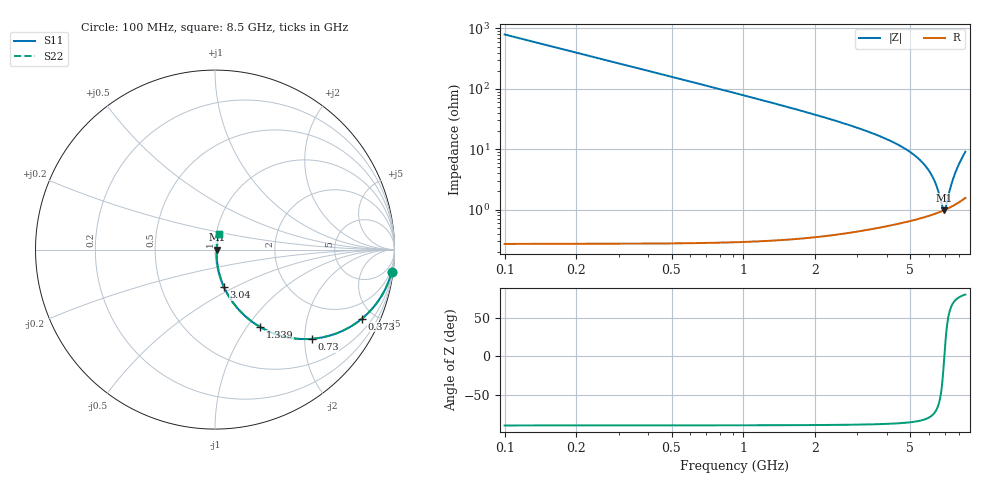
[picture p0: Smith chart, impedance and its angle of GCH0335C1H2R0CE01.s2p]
!Murata Part Number: GCH0335C1H2R0CE01
!These Parameters are Measured in Series Mode Connection
!Data Generated on Mar 13, 2026
!  o--ll--o
!Port1  Port2
!  o------o
!Operation Temp=25[degC], DC Bias Voltage=0[V]
!Freq. Start=100[MHz] Stop=9[GHz] 401[Steps]
# Hz S RI R 50
!Freq.(Hz) S11(Real) S11(Imag) S21(Real) S21(Imag) S12(Real) S12(Imag) S22(Real) S22(Imag)
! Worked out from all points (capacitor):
!   401 points, 100 MHz to 8.5 GHz, reference 50 ohm
!   read as one part in series: C = 2 pF near 142 MHz
!   lowest |Z| = 979 mohm at 6.925 GHz (marker M1)
!   series resonance near 6.94 GHz, so ESL is about 260 pH
!   S11 on the Smith chart (normalised r, x): 100 MHz: 1, -16; 373 MHz: 1.01, -4.26; 730 MHz: 1.01, -2.16; 1.339 GHz: 1.01, -1.15; 3.04 GHz: 1.01, -0.44; 8.5 GHz: 1.03, +0.18
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1e8  0.9844 -0.1237  0.0156 0.1237  0.0156 0.1237  0.9844 -0.1237
2.26e8  0.9251 -0.2629  0.0749 0.2629  0.0749 0.2629  0.9251 -0.2629
3.73e8  0.8189 -0.3845  0.1811 0.3845  0.1811 0.3845  0.8189 -0.3845
5.41e8  0.6816 -0.4649  0.3184 0.4649  0.3184 0.4649  0.6816 -0.4649
7.3e8  0.5387 -0.4972  0.4613 0.4972  0.4613 0.4972  0.5387 -0.4972
1.024e9  0.3691 -0.4807  0.6309 0.4807  0.6309 0.4807  0.3691 -0.4807
1.339e9  0.2511 -0.431  0.7489 0.431  0.7489 0.431  0.2511 -0.431
1.507e9  0.2072 -0.4022  0.7928 0.4022  0.7928 0.4022  0.2072 -0.4022
2.095e9  0.1133 -0.312  0.8867 0.312  0.8867 0.312  0.1133 -0.312
2.914e9  0.0561 -0.2212  0.9439 0.2212  0.9439 0.2212  0.0561 -0.2212
3.04e9  0.0508 -0.2101  0.9492 0.2101  0.9492 0.2101  0.0508 -0.2101
4.3e9  0.0212 -0.1236  0.9788 0.1236  0.9788 0.1236  0.0212 -0.1236
5.707e9  0.0104 -0.0548  0.9896 0.0548  0.9896 0.0548  0.0104 -0.0548
6.316e9  0.00918 -0.0279  0.9908 0.0279  0.9908 0.0279  0.00918 -0.0279
6.547e9  0.00916 -0.0177  0.9908 0.0177  0.9908 0.0177  0.00916 -0.0177
6.82e9  0.00946 -0.00549  0.9905 0.00549  0.9905 0.00549  0.00946 -0.00549
6.925e9  0.00967 -0.000691  0.9903 0.000691  0.9903 0.000691  0.00967 -0.000691
7.009e9  0.00989 0.00319  0.9901 -0.00319  0.9901 -0.00319  0.00989 0.00319
7.114e9  0.0102 0.00811  0.9898 -0.00811  0.9898 -0.00811  0.0102 0.00811
7.387e9  0.0114 0.0213  0.9886 -0.0213  0.9886 -0.0213  0.0114 0.0213
7.66e9  0.0131 0.0353  0.9869 -0.0353  0.9869 -0.0353  0.0131 0.0353
8.5e9  0.023 0.0863  0.977 -0.0863  0.977 -0.0863  0.023 0.0863
